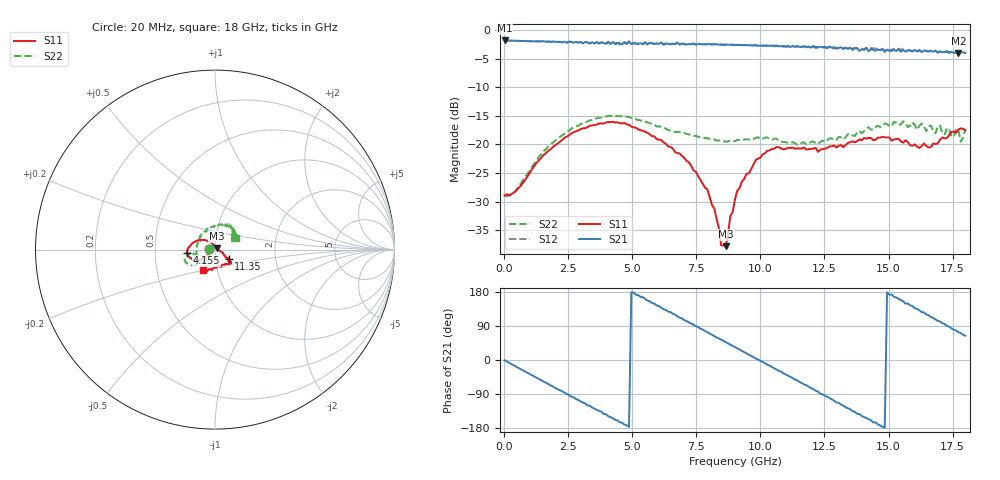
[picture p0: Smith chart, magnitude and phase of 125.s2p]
!Agilent Technologies,N5230A,US43500223,A.07.50.48
!Agilent N5230A: A.07.50.48
!Date: Tuesday, January 12, 2016 20:47:00
!Correction: S11(Full 2 Port(1,2))
!S21(Full 2 Port(1,2))
!S12(Full 2 Port(1,2))
!S22(Full 2 Port(1,2))
!S2P File: Measurements: S11, S21, S12, S22:
# Hz S  dB  R 50
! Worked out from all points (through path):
!   201 points, 20 MHz to 18 GHz, reference 50 ohm
!   highest |S21| = -1.79 dB at 20 MHz (marker M1); lowest = -4.0 dB at 17.73 GHz (marker M2)
!   group delay of S21, straight-line fit = 101 ps
!   lowest |S11| = -37.8 dB at 8.65 GHz (marker M3), VSWR 1.03, Z = 51.1 + j0.646 ohm
!   |S11| at or under -10 dB: start of sweep to end of sweep
!   |S22| runs from -29.1 to -14.9 dB; largest |S21 - S12| = 0.033
!   S11 on the Smith chart (normalised r, x): 20 MHz: 0.93, +0.00; 4.155 GHz: 0.73, -0.03; 11.35 GHz: 1.16, -0.12; 18 GHz: 0.85, -0.20
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2e7  -28.91 178.5  -1.79 -0.8  -1.80 -0.8  -28.89 178.2
1.5483e9  -21.80 -141.2  -1.93 -57.1  -1.95 -57.3  -21.15 -133.1
2.3574e9  -18.83 -149.2  -2.01 -86.2  -2.05 -86.1  -18.09 -137.7
3.0766e9  -17.17 -157.3  -2.30 -112.5  -2.24 -112.4  -16.25 -145.0
4.1554e9  -16.09 -173.4  -2.40 -150.6  -2.37 -150.8  -15.00 -156.5
4.8746e9  -16.53 175.0  -1.94 -176.5  -2.12 -176.0  -15.15 -163.6
6.0433e9  -19.13 152.3  -2.40 142.3  -2.49 142.0  -16.83 -171.1
7.3918e9  -24.55 129.4  -2.32 92.7  -2.39 92.7  -18.51 -167.9
7.9312e9  -27.84 113.6  -2.47 73.5  -2.49 73.3  -18.89 -163.5
8.4706e9  -37.67 71.9  -2.49 53.5  -2.53 53.5  -19.30 -157.6
8.6504e9  -37.79 29.3  -2.50 47.2  -2.55 46.8  -19.50 -155.5
9.01e9  -29.59 -20.1  -2.59 34.1  -2.57 33.8  -19.43 -150.5
1.01787e10  -21.52 -37.9  -2.68 -8.2  -2.73 -8.6  -18.80 -150.9
1.13474e10  -20.72 -34.9  -2.91 -51.4  -2.88 -50.8  -19.77 178.4
1.20666e10  -20.70 -33.2  -2.74 -76.8  -2.91 -77.8  -19.50 152.0
1.28757e10  -20.15 -36.5  -2.97 -107.1  -3.13 -107.1  -19.19 126.5
1.37747e10  -19.41 -40.6  -3.14 -141.9  -3.20 -141.4  -17.93 99.9
1.50333e10  -18.77 -40.3  -3.62 172.3  -3.53 173.0  -16.80 64.6
1.64717e10  -20.24 -74.0  -3.58 120.2  -3.65 118.8  -17.69 43.7
1.77303e10  -17.34 -115.7  -4.00 73.4  -3.98 72.5  -17.59 24.0
1.78202e10  -17.18 -116.1  -3.91 71.0  -4.04 70.3  -19.54 24.7
1.8e10  -17.49 -119.6  -3.96 64.1  -4.03 62.9  -17.37 28.4
